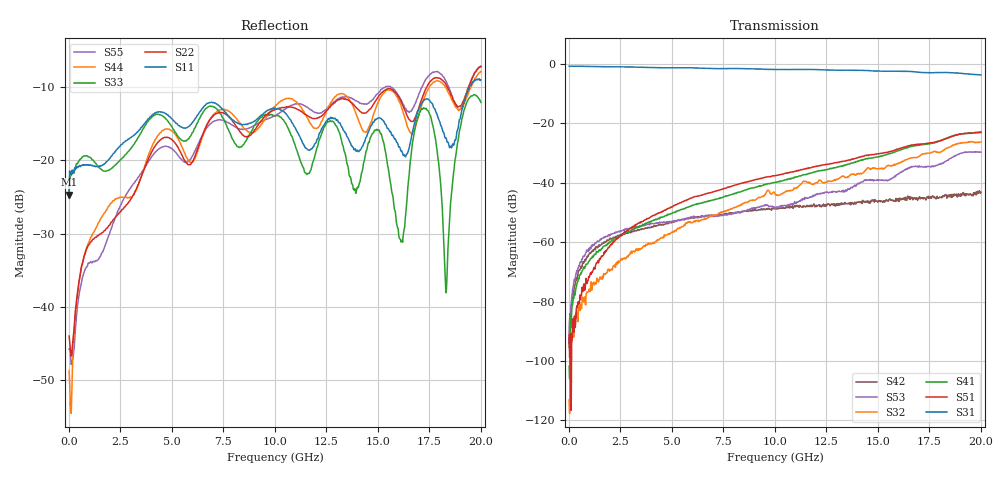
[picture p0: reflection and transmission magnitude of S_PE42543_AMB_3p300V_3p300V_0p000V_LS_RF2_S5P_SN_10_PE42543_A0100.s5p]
!Agilent Technologies,N5230C,MY49001593,A.09.33.09
!Agilent N5230C: A.09.33.09
!Date: Friday, March 21, 2014 07:23:05
!Correction: S11(Full 5 Port(1,2,3,5,6))
!S12(Full 5 Port(1,2,3,5,6))
!S13(Full 5 Port(1,2,3,5,6))
!S15(Full 5 Port(1,2,3,5,6))
!S16(Full 5 Port(1,2,3,5,6))
!S21(Full 5 Port(1,2,3,5,6))
!S22(Full 5 Port(1,2,3,5,6))
!S23(Full 5 Port(1,2,3,5,6))
!S25(Full 5 Port(1,2,3,5,6))
!S26(Full 5 Port(1,2,3,5,6))
!S31(Full 5 Port(1,2,3,5,6))
!S32(Full 5 Port(1,2,3,5,6))
!S33(Full 5 Port(1,2,3,5,6))
!S35(Full 5 Port(1,2,3,5,6))
!S36(Full 5 Port(1,2,3,5,6))
!S51(Full 5 Port(1,2,3,5,6))
!S52(Full 5 Port(1,2,3,5,6))
!S53(Full 5 Port(1,2,3,5,6))
!S55(Full 5 Port(1,2,3,5,6))
!S56(Full 5 Port(1,2,3,5,6))
!S61(Full 5 Port(1,2,3,5,6))
!S62(Full 5 Port(1,2,3,5,6))
!S63(Full 5 Port(1,2,3,5,6))
!S65(Full 5 Port(1,2,3,5,6))
!S66(Full 5 Port(1,2,3,5,6))
!S5P File: Measurements: <S11,S12,S13,S15,S16>,
!<S21,S22,S23,S25,S26>,
!<S31,S32,S33,S35,S36>,
!<S51,S52,S53,S55,S56>,
!<S61,S62,S63,S65,S66>:
# Hz S  dB  R 50
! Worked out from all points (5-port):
!   801 points, 10 MHz to 20 GHz, reference 50 ohm
!   strongest paths, dB at 10 MHz, 5.008 GHz, 10.01 GHz, 15 GHz, 20 GHz:
!     S31: -0.8, -1.3, -1.9, -2.4, -3.7
!     S51: -91.3, -48.1, -37.6, -30.3, -23.1
!     S41: -101.7, -50.2, -39.9, -31.3, -22.9
!     S32: -113.0, -56.7, -43.6, -35.3, -26.3
!     S53: -94.1, -53.1, -48.2, -39.0, -29.7
!     S42: -95.4, -53.0, -48.7, -46.5, -43.2
!   lowest |S11| = -24.7 dB at 10 MHz (marker M1), VSWR 1.12, Z = 55.8 - j2.01 ohm
!   |S11| at or under -10 dB: start of sweep to 19.45 GHz
